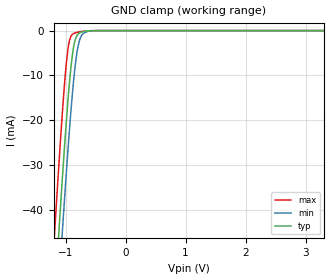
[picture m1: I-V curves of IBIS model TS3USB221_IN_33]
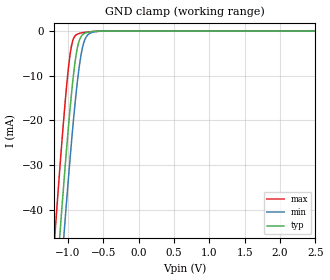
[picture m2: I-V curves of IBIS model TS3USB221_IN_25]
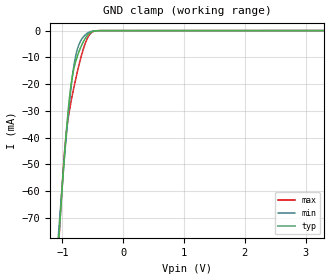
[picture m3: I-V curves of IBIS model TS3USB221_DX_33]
| TEXAS INSTRUMENTS INCORPORATED
| Standard Linear and Logic Group
| IBIS Model of TS3USB221
| HIGH-SPEED USB 2.0 (480-Mbps) 1:2 MULIPLEXER/DEMULTIPLEXER SWITCH
| WITH SINGLE ENABLE
| This file contains package information for the following:
|  LGA 10-pin (RSE) package as [Component] TS3USB221_RSE
|  QFN 10-pin (DRC) package as [Component] TS3USB221_DRC
| This device can be powered at the following Vccs:
|  3.3 volt Vcc
|  2.5 volt Vcc
| This file provides unique models under the [Model Selector] for each Vcc.
| For operation at a specific Vcc, select the appropriate model after each
| [Model Selector] keyword.
[IBIS Ver]   3.2
[Comment char]  |_char
[File Name]   ts3usb221.ibs
[File Rev]   1.2 | x_die
[Date]   March 19, 2013
[Source]   Data created from TI-SPICE simulations at TI-SLL.
[Notes]   The following is an IBIS list for the TS3USB221.
   Please contact sllibis@ti.com with questions and
   comments concerning SLL IBIS models.
   - FILE REV HISTORY
   - 1.1 Release IBIS file on 12/14/06
   - Power clamp data deleted as there is no power-clamp diode.
   - 1.2, add package model for QFN on 3/19/13
[Disclaimer] Property of Texas Instruments Incorporated.  Unauthorized
   reproduction and/or distribution is strictly prohibited.
   This product is protected under copyright law.
   Created  2006, (C) Copyright  2006, Texas Instruments
   Incorporated, All Rights Reserved
   UNLESS THERE IS A SIGNED, WRITTEN AGREEMENT TO THE
   CONTRARY, TEXAS INSTRUMENTS (TI) IS PROVIDING THE IBIS
   MODELS  AND WITHOUT ANY WARRANTY, EXPRESSED OR
   IMPLIED.  TI assumes no liability for:
   1) the accuracy of the IBIS models provided to your
   company;
   2) the proper functioning of these IBIS Models in your
   design or for any resulting applications; or
   3) infringement of patents, copyrights or intellectual
   property rights resulting from your use of these IBIS
   models.
   TI provides IBIS Models as a service to our customers.
   You and your company shall not distribute, sell or give
   these models to anyone else without prior written
   permission from TI.
   TI reserves the right to make changes to our products or
   to discontinue any semiconductor product or service
   without notice, and advises our customers to obtain the
   latest version of relevant information to verify, before
   placing orders, that the information being relied on is
   current.
   Please be aware that your receipt and use of the IBIS
   information provided shall serve as acceptance of these
   terms and conditions.  If you do not accept these terms,
   you should return or destroy the IBIS models and any
   other accompanying information immediately.
| Component TS3USB221_RSE 10-PIN LGA
[Component]   TS3USB221_RSE
[Manufacturer]   Texas Instruments, Inc.
[Package]
|   typ   min   max
R_pkg   1.700e-02   1.500e-02   2.200e-02
L_pkg   5.570e-10   4.830e-10   6.520e-10
C_pkg   1.440e-13   1.050e-13   1.870e-13
[Pin]   signal_name   model_name   R_pin   L_pin   C_pin
1   1DP   TS3USB221_XDX   1.600e-02   4.830e-10   1.100e-13
2   1DM   TS3USB221_XDX   1.500e-02   5.130e-10   1.860e-13
3   2DP   TS3USB221_XDX   1.800e-02   5.860e-10   1.870e-13
4   2DM   TS3USB221_XDX   2.200e-02   6.520e-10   1.180e-13
5   GND   GND   1.600e-02   5.500e-10   1.250e-13
6   NOE   TS3USB221_IN   1.600e-02   4.830e-10   1.050e-13
7   DM   TS3USB221_DX   1.500e-02   5.150e-10   1.820e-13
8   DP   TS3USB221_DX   1.700e-02   5.790e-10   1.870e-13
9   S   TS3USB221_IN   2.200e-02   6.360e-10   1.170e-13
10   VCC   POWER   1.700e-02   5.710e-10   1.280e-13
| Component TS3USB221_DRC 10-PIN QFN
[Component]   TS3USB221_DRC
[Manufacturer]   Texas Instruments, Inc.
[Package]
|   typ   min   max
R_pkg   0.090355   0.08685   0.10179
L_pkg   1.26614n   1.21776n   1.44522n
C_pkg   0.17341p   0.15515p   0.17814p
[Pin]   signal_name   model_name   R_pin   L_pin   C_pin
1   1DP   TS3USB221_XDX   0.09817   1.39142n   0.16724p
2   1DM   TS3USB221_XDX   0.08944   1.25699n   0.17814p
3   2DP   TS3USB221_XDX   0.08685   1.21826n   0.17549p
4   2DM   TS3USB221_XDX   0.09136   1.28519n   0.17723p
5   GND   GND   0.10179   1.44522n   0.16712p
6   NOE   TS3USB221_IN   0.08819   1.23652n   0.15515p
7   DM   TS3USB221_DX   0.09127   1.27529n   0.17552p
8   DP   TS3USB221_DX   0.08742   1.21776n   0.17314p
9   S   TS3USB221_IN   0.08757   1.22069n   0.17368p
10   VCC   POWER   0.09275   1.30332n   0.16113p
[Series Switch Groups]
| Function Group States
On  1 /   | DP->1DP S LOW
   | DM->1DM S LOW
On  2 /   | DP->2DP S HIGH
   | DM->2DM S HIGH
On  3 /   | 1DP->DP S LOW
   | 1DM->DM S LOW
On  4 /   | 2DP->DP S HIGH
   | 2DM->DM S HIGH
On  1 2 3 4 /   | NOE LOW
Off 1 2 3 4 /   | NOE HIGH
[Series Pin Mapping]   pin_2   model_name   function_table_group
8   1   TS3USB221_DX_33_S   1
| 8   1   TS3USB221_DX_25_S   1
7   2   TS3USB221_DX_33_S   1
| 7   2   TS3USB221_DX_25_S   1
8   3   TS3USB221_DX_33_S   2
| 8   3   TS3USB221_DX_25_S   2
7   4   TS3USB221_DX_33_S   2
| 7   4   TS3USB221_DX_25_S   2
1   8   TS3USB221_XDX_33_S   3
| 1   8   TS3USB221_XDX_25_S   3
2   7   TS3USB221_XDX_33_S   3
| 2   7   TS3USB221_XDX_25_S   3
3   8   TS3USB221_XDX_33_S   4
| 3   8   TS3USB221_XDX_25_S   4
4   7   TS3USB221_XDX_33_S   4
| 4   7   TS3USB221_XDX_25_S   4
| Model TS3USB221_IN
[Model Selector]   TS3USB221_IN
TS3USB221_IN_33   3.3 volt Vcc
TS3USB221_IN_25   2.5 volt Vcc
| Model TS3USB221_DX
[Model Selector]   TS3USB221_DX
TS3USB221_DX_33   3.3 volt Vcc
TS3USB221_DX_25   2.5 volt Vcc
| Model TS3USB221_XDX
[Model Selector]   TS3USB221_XDX
TS3USB221_XDX_33   3.3 volt Vcc
TS3USB221_XDX_25   2.5 volt Vcc
[Model]   TS3USB221_DX_33_S
Model_type  Series_switch
| variable   typ   min   max
C_comp   0   0   0
[Temperature Range]   40   100   -40
| Ambient temperature   25   85   -40
[Voltage range]   3.3   3   3.6
[On]
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[Off]
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[Model]   TS3USB221_DX_25_S
Model_type  Series_switch
| variable   typ   min   max
C_comp   0   0   0
[Temperature Range]   40   100   -40
| Ambient temperature   25   85   -40
[Voltage range]   2.5   2.3   2.7
[On]
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[Off]
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[Model]   TS3USB221_XDX_33_S
Model_type  Series_switch
| variable   typ   min   max
C_comp   0   0   0
[Temperature Range]   40   100   -40
| Ambient temperature   25   85   -40
[Voltage range]   3.3   3   3.6
[On]
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[Off]
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[Model]   TS3USB221_XDX_25_S
Model_type  Series_switch
| variable   typ   min   max
C_comp   0   0   0
[Temperature Range]   40   100   -40
| Ambient temperature   25   85   -40
[Voltage range]   2.5   2.3   2.7
[On]
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[Off]
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| Models and submodels in the file (10): TS3USB221_IN_33 (Input), TS3USB221_IN_25 (Input), TS3USB221_DX_33_S (Series_switch), TS3USB221_DX_33 (Terminator), TS3USB221_DX_25_S (Series_switch), TS3USB221_DX_25 (Terminator), TS3USB221_XDX_33_S (Series_switch), TS3USB221_XDX_33 (Terminator), TS3USB221_XDX_25_S (Series_switch), TS3USB221_XDX_25 (Terminator)
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[Model]   TS3USB221_IN_33
Model_type  Input
Vinl=0.825
Vinh=1.518
| variable   typ   min   max
C_comp   1.34pF   0.96pF   1.59pF
[Temperature Range]   40   100   -40
| Ambient temperature   25   85   -40
[Voltage range]   3.3   3   3.6
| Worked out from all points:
|   GND clamp passes 1 mA (typ) near -0.80 V on its own axis
[GND Clamp]
| TS3USB221_IN_33
|   Voltage   I(typ)   I(min)   I(max)
-3.3V     -560.9mA   -570.2mA   -549.9mA
-1.18V    -59.71mA   -71.83mA   -44.66mA
-1.115V   -45.76mA   -57.84mA   -30.76mA
-1.05V    -32.37mA   -44.28mA   -17.83mA
-995mV    -21.8mA    -33.31mA   -8.515mA
-955mV    -14.83mA   -25.76mA   -3.752mA
-905mV    -7.595mA   -17.09mA   -1.186mA
-860mV    -3.269mA   -10.41mA   -636.9uA
-810mV    -1.123mA   -4.908mA   -410.2uA
-765mV    -512uA     -2.083mA   -285.4uA
-635mV    -85.97uA   -202.3uA   -73.27uA
3.3V      132.3pA    457.5pA    41.25pA
[Model]   TS3USB221_IN_25
Model_type  Input
Vinl=0.625
Vinh=1.15
| variable   typ   min   max
C_comp   1.35pF   0.96pF   1.61pF
[Temperature Range]   40   100   -40
| Ambient temperature   25   85   -40
[Voltage range]   2.5   2.3   2.7
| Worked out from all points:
|   GND clamp passes 1 mA (typ) near -0.80 V on its own axis
[GND Clamp]
| TS3USB221_IN_25
|   Voltage   I(typ)   I(min)   I(max)
-2.5V     -368.7mA   -379mA     -356.5mA
-1.18V    -59.71mA   -71.83mA   -44.66mA
-1.105V   -43.65mA   -55.72mA   -28.69mA
-1.055V   -33.38mA   -45.31mA   -18.77mA
-1V       -22.72mA   -34.28mA   -9.257mA
-960mV    -15.66mA   -26.67mA   -4.215mA
-925mV    -10.24mA   -20.43mA   -1.817mA
-875mV    -4.439mA   -12.48mA   -751uA
-825mV    -1.534mA   -6.304mA   -464.7uA
-775mV    -597.4uA   -2.545mA   -309uA
-650mV    -107.2uA   -256.9uA   -90.81uA
2.5V      97.49pA    374.5pA    30.7pA
[Model]   TS3USB221_DX_33
Model_type  Terminator
| variable   typ   min   max
C_comp   3.36pF   3.11pF   3.63pF
| C_tri-state   3.36pF   3.11pF   3.63pF
[Temperature Range]   40   100   -40
| Ambient temperature   25   85   -40
[Voltage range]   3.3   3   3.6
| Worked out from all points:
|   GND clamp passes 1 mA (typ) near -0.55 V on its own axis
[GND Clamp]
| TS3USB221_DX_33
|   Voltage   I(typ)   I(min)   I(max)
-3.3V     -1.11A     -970.4mA   -1.236A
-1.06V    -78.09mA   -74.57mA   -79.3mA
-1.05V    -74.53mA   -71.53mA   -75.24mA
-985mV    -52.56mA   -52.54mA   -51.32mA
-940mV    -38.97mA   -40.33mA   -39.05mA
-890mV    -26.38mA   -28.08mA   -30.54mA
-845mV    -18.27mA   -18.73mA   -25.01mA
-800mV    -13.1mA    -11.62mA   -20.06mA
-745mV    -8.945mA   -6.252mA   -14.49mA
-570mV    -1.335mA   -717.6uA   -2.079mA
-370mV    -14.47uA   -10.28uA   -8.844uA
3.3V      836.7pA    1.391nA    104pA
